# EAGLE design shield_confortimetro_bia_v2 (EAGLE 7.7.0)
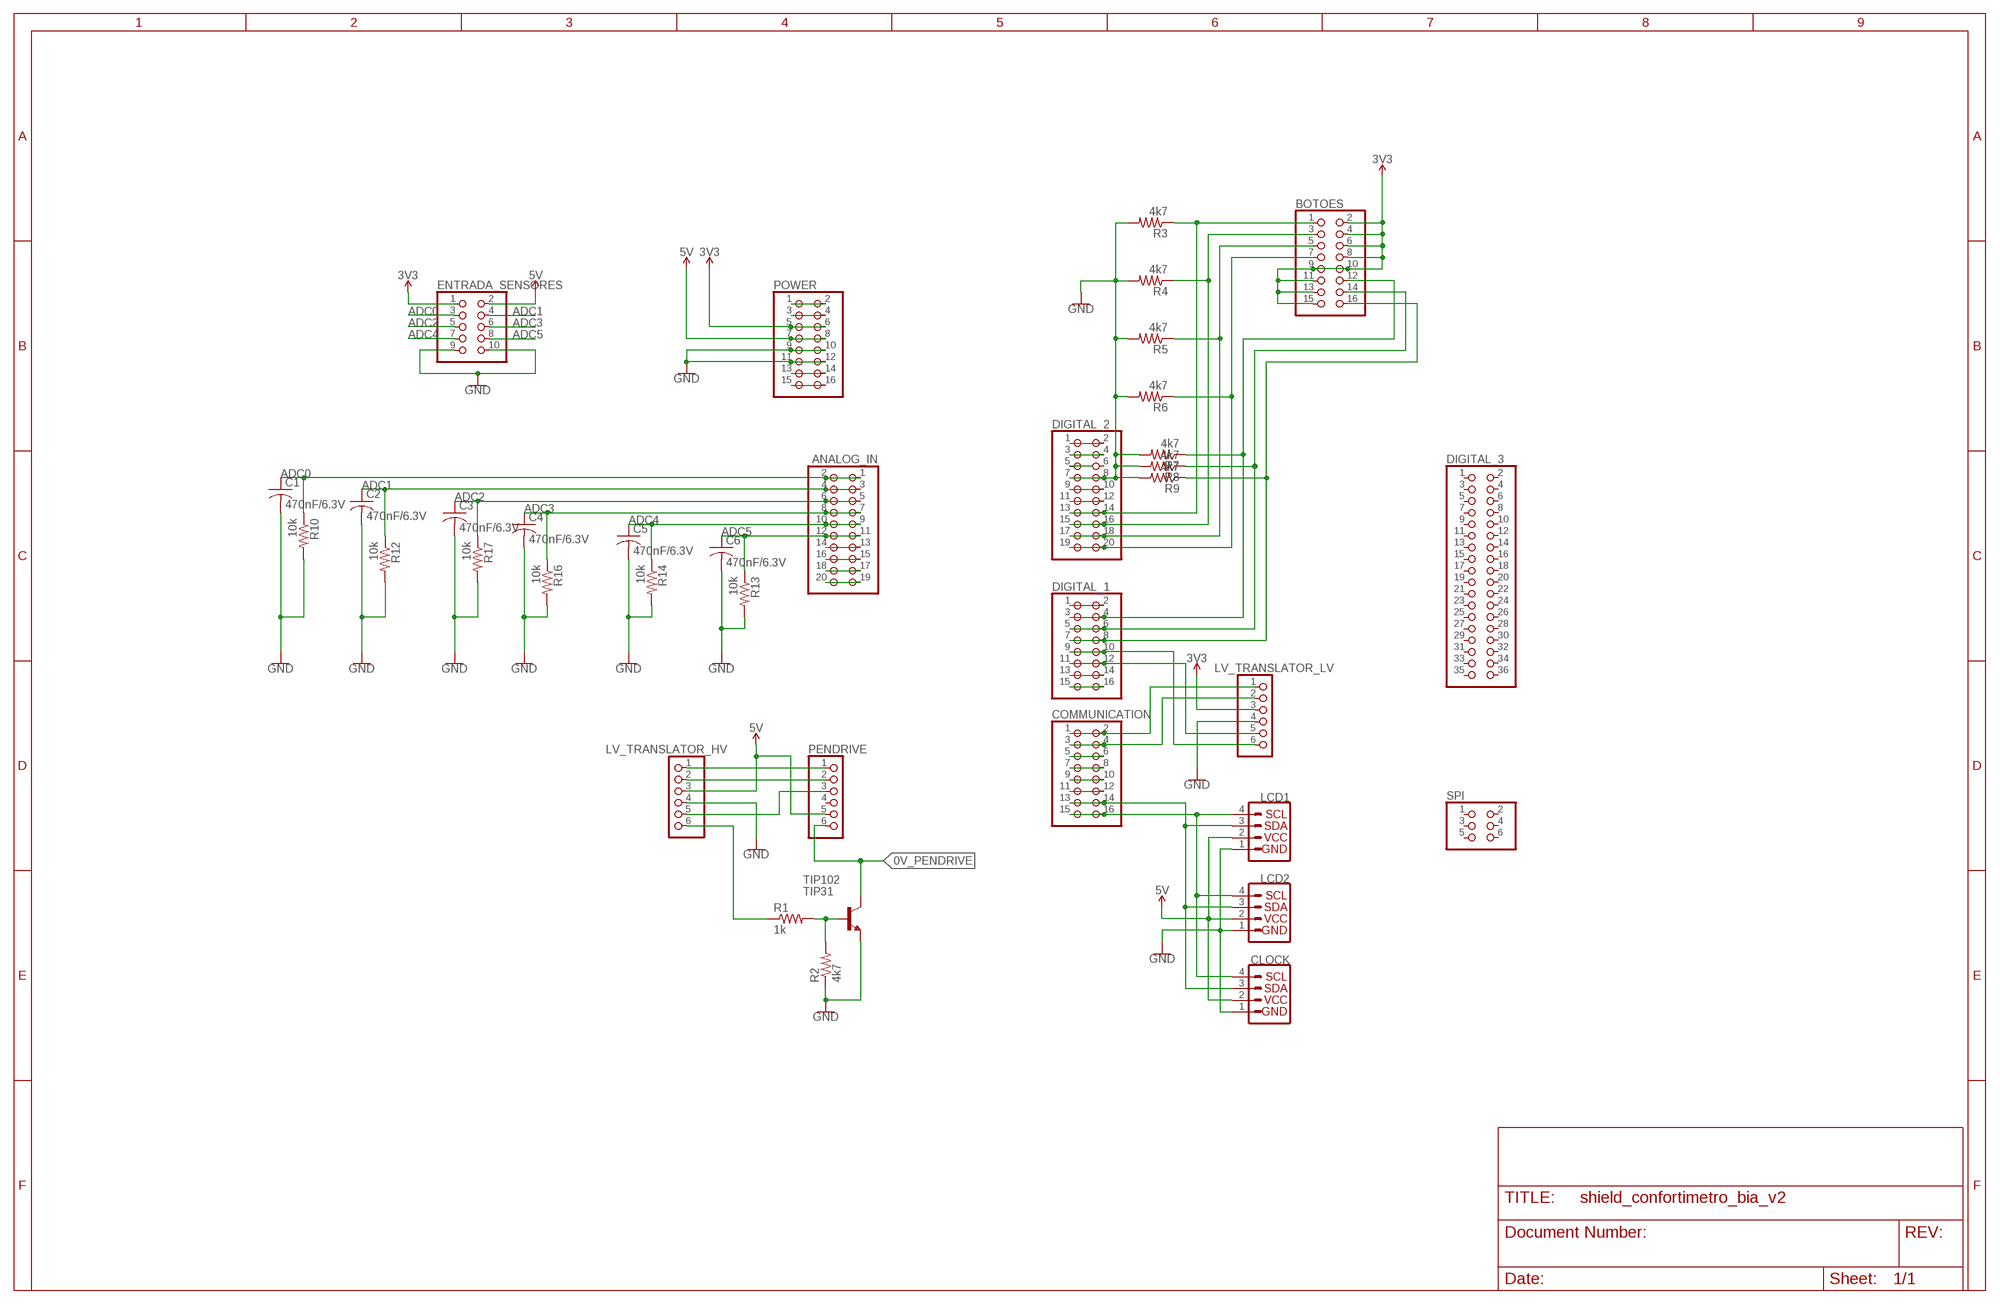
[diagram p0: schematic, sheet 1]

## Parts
ANALOG_IN  PINHD-2X10  [2X10]
BOTOES  PINHD-2X8  [2X08]
C1  470nF/6.3V  C-US050-030X075  [C050-030X075]
C2  470nF/6.3V  C-US050-030X075  [C050-030X075]
C3  470nF/6.3V  C-US050-030X075  [C050-030X075]
C4  470nF/6.3V  C-US050-030X075  [C050-030X075]
C5  470nF/6.3V  C-US050-030X075  [C050-030X075]
C6  470nF/6.3V  C-US050-030X075  [C050-030X075]
CLOCK  I2C_STANDARD  [1X04]
COMMUNICATION  PINHD-2X8  [2X08]
DIGITAL_1  PINHD-2X8  [2X08]
DIGITAL_2  PINHD-2X10  [2X10]
DIGITAL_3  PINHD-2X18  [2X18]
ENTRADA_SENSORES  PINHD-2X5  [2X05]
LCD1  I2C_STANDARD  [1X04]
LCD2  I2C_STANDARD  [1X04]
LV_TRANSLATOR_HV  PINHD-1X6  [1X06]
LV_TRANSLATOR_LV  PINHD-1X6  [1X06]
PENDRIVE  PINHD-1X6  [1X06]
POWER  PINHD-2X8  [2X08]
R1  1k  R-US_0309/12  [0309/12]
R2  4k7  R-US_0309/12  [0309/12]
R3  4k7  R-US_0309/12  [0309/12]
R4  4k7  R-US_0309/12  [0309/12]
R5  4k7  R-US_0309/12  [0309/12]
R6  4k7  R-US_0309/12  [0309/12]
R7  4k7  R-US_0309/12  [0309/12]
R8  4k7  R-US_0309/12  [0309/12]
R9  4k7  R-US_0309/12  [0309/12]
R10  10k  R-US_0309/12  [0309/12]
R12  10k  R-US_0309/12  [0309/12]
R13  10k  R-US_0309/12  [0309/12]
R14  10k  R-US_0309/12  [0309/12]
R16  10k  R-US_0309/12  [0309/12]
R17  10k  R-US_0309/12  [0309/12]
SPI  PINHD-2X3  [2X03]
TIP102  TIP31  [TO220]

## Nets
0V_PENDRIVE: PENDRIVE.6 TIP102.2(C)
ADC0: ANALOG_IN.1 ANALOG_IN.2 C1.1 ENTRADA_SENSORES.3 R10.1
ADC1: ANALOG_IN.3 ANALOG_IN.4 C2.1 ENTRADA_SENSORES.4 R12.1
ADC2: ANALOG_IN.5 ANALOG_IN.6 C3.1 ENTRADA_SENSORES.5 R17.1
ADC3: ANALOG_IN.7 ANALOG_IN.8 C4.1 ENTRADA_SENSORES.6 R16.1
ADC4: ANALOG_IN.9 ANALOG_IN.10 C5.1 ENTRADA_SENSORES.7 R14.1
ADC5: ANALOG_IN.11 ANALOG_IN.12 C6.1 ENTRADA_SENSORES.8 R13.1
GND: C1.2 C2.2 C3.2 C4.2 C5.2 C6.2 CLOCK.1 DIGITAL_2.7 DIGITAL_2.8 ENTRADA_SENSORES.9 ENTRADA_SENSORES.10 LCD1.1 LCD2.1 LV_TRANSLATOR_HV.4 LV_TRANSLATOR_LV.4 POWER.9 POWER.10 POWER.11 POWER.12 R2.1 R3.2 R4.2 R5.2 R6.2 R7.2 R8.2 R9.2 R10.2 R12.2 R13.2 R14.2 R16.2 R17.2 TIP102.3(E)
N$1: CLOCK.3 COMMUNICATION.13 COMMUNICATION.14 LCD1.3 LCD2.3
N$2: CLOCK.4 COMMUNICATION.15 COMMUNICATION.16 LCD1.4 LCD2.4
N$3: COMMUNICATION.1 COMMUNICATION.2 LV_TRANSLATOR_LV.1
N$4: COMMUNICATION.3 COMMUNICATION.4 LV_TRANSLATOR_LV.2
N$5: DIGITAL_1.9 DIGITAL_1.10 LV_TRANSLATOR_LV.6
N$6: DIGITAL_1.11 DIGITAL_1.12 LV_TRANSLATOR_LV.5
N$7: LV_TRANSLATOR_HV.1 PENDRIVE.1
N$8: LV_TRANSLATOR_HV.2 PENDRIVE.2
N$9: LV_TRANSLATOR_HV.5 PENDRIVE.3
N$10: R1.2 R2.2 TIP102.1(B)
N$11: LV_TRANSLATOR_HV.6 R1.1
N$12: BOTOES.12 DIGITAL_1.3 DIGITAL_1.4 R7.1
N$13: BOTOES.14 DIGITAL_1.5 DIGITAL_1.6 R8.1
N$14: BOTOES.16 DIGITAL_1.7 DIGITAL_1.8 R9.1
N$15: BOTOES.7 DIGITAL_2.19 DIGITAL_2.20 R6.1
N$16: BOTOES.5 DIGITAL_2.17 DIGITAL_2.18 R5.1
N$17: BOTOES.3 DIGITAL_2.15 DIGITAL_2.16 R4.1
N$18: BOTOES.1 DIGITAL_2.13 DIGITAL_2.14 R3.1
N$19: POWER.1 POWER.2
N$20: POWER.3 POWER.4
N$21: POWER.13 POWER.14
N$22: POWER.15 POWER.16
N$23: ANALOG_IN.13 ANALOG_IN.14
N$24: ANALOG_IN.15 ANALOG_IN.16
N$25: DIGITAL_2.1 DIGITAL_2.2
N$26: DIGITAL_2.3 DIGITAL_2.4
N$27: DIGITAL_2.5
N$29: DIGITAL_2.9 DIGITAL_2.10
N$30: DIGITAL_2.11 DIGITAL_2.12
N$31: DIGITAL_1.1 DIGITAL_1.2
N$32: DIGITAL_1.13 DIGITAL_1.14
N$33: DIGITAL_1.15 DIGITAL_1.16
N$34: COMMUNICATION.5 COMMUNICATION.6
N$35: COMMUNICATION.7 COMMUNICATION.8
N$36: COMMUNICATION.9 COMMUNICATION.10
N$37: COMMUNICATION.11 COMMUNICATION.12
N$38: ANALOG_IN.17 ANALOG_IN.18
N$39: ANALOG_IN.19 ANALOG_IN.20
VCC_3V3: BOTOES.2 BOTOES.4 BOTOES.6 BOTOES.8 BOTOES.9 BOTOES.10 BOTOES.11 BOTOES.13 BOTOES.15 ENTRADA_SENSORES.1 LV_TRANSLATOR_LV.3 POWER.5 POWER.6 ; supply symbol labelled 3V3
VCC_5V: CLOCK.2 ENTRADA_SENSORES.2 LCD1.2 LCD2.2 LV_TRANSLATOR_HV.3 PENDRIVE.5 POWER.7 POWER.8 ; supply symbol labelled 5V
Unconnected: DIGITAL_2.6 DIGITAL_3.1 DIGITAL_3.2 DIGITAL_3.3 DIGITAL_3.4 DIGITAL_3.5 DIGITAL_3.6 DIGITAL_3.7 DIGITAL_3.8 DIGITAL_3.9 DIGITAL_3.10 DIGITAL_3.11 DIGITAL_3.12 DIGITAL_3.13 DIGITAL_3.14 DIGITAL_3.15 DIGITAL_3.16 DIGITAL_3.17 DIGITAL_3.18 DIGITAL_3.19 DIGITAL_3.20 DIGITAL_3.21 DIGITAL_3.22 DIGITAL_3.23 DIGITAL_3.24 DIGITAL_3.25 DIGITAL_3.26 DIGITAL_3.27 DIGITAL_3.28 DIGITAL_3.29 DIGITAL_3.30 DIGITAL_3.31 DIGITAL_3.32 DIGITAL_3.33 DIGITAL_3.34 DIGITAL_3.35 DIGITAL_3.36 PENDRIVE.4 SPI.1 SPI.2 SPI.3 SPI.4 SPI.5 SPI.6

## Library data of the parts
ANALOG_IN = SparkFun-Retired:PINHD-2X10: PIN HEADER
BOTOES COMMUNICATION DIGITAL_1 POWER = pinhead:PINHD-2X8: PIN HEADER
C1-C6 = adafruit:C-US: CAPACITOR, American symbol
CLOCK LCD1 LCD2 = SparkFun-Connectors:I2C_STANDARD: SparkFun I2C Standard Pinout Header SparkFun has standardized on a pinout for all I2C based sensor breakouts. This pinout allows I2C boards to be plugged directly into the headers on Arduino Uno compatible boards, and to be daisy chained easily. Example SparkFun Products: SparkFun Atmospheric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
DIGITAL_2 = pinhead:PINHD-2X10: PIN HEADER
DIGITAL_3 = pinhead:PINHD-2X18: PIN HEADER
ENTRADA_SENSORES = pinhead:PINHD-2X5: PIN HEADER
LV_TRANSLATOR_HV LV_TRANSLATOR_LV PENDRIVE = adafruit:PINHD-1X6: PIN HEADER
R1-R10 R12-R14 R16 R17 = adafruit:R-US_: RESISTOR, American symbol
SPI = pinhead:PINHD-2X3: PIN HEADER
TIP102 = transistor:TIP31: NPN Transistor Medium Power Linear Switching Applications Source: http://onsemi.com

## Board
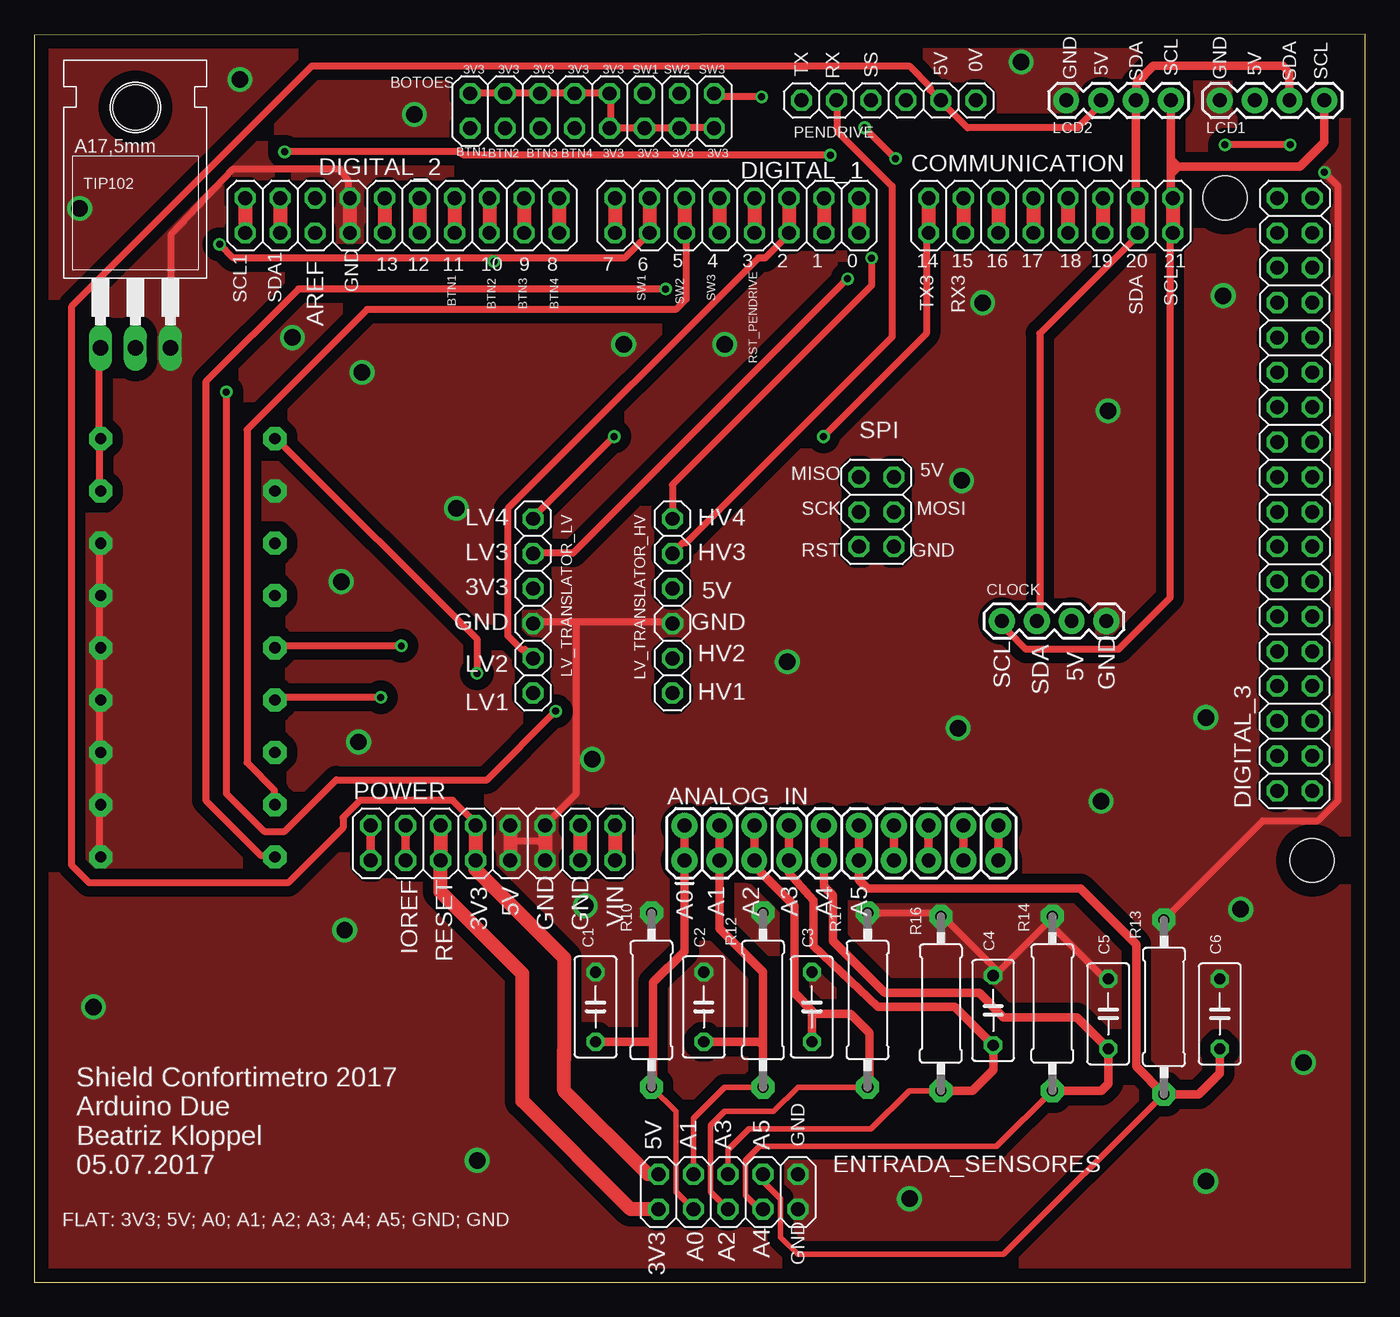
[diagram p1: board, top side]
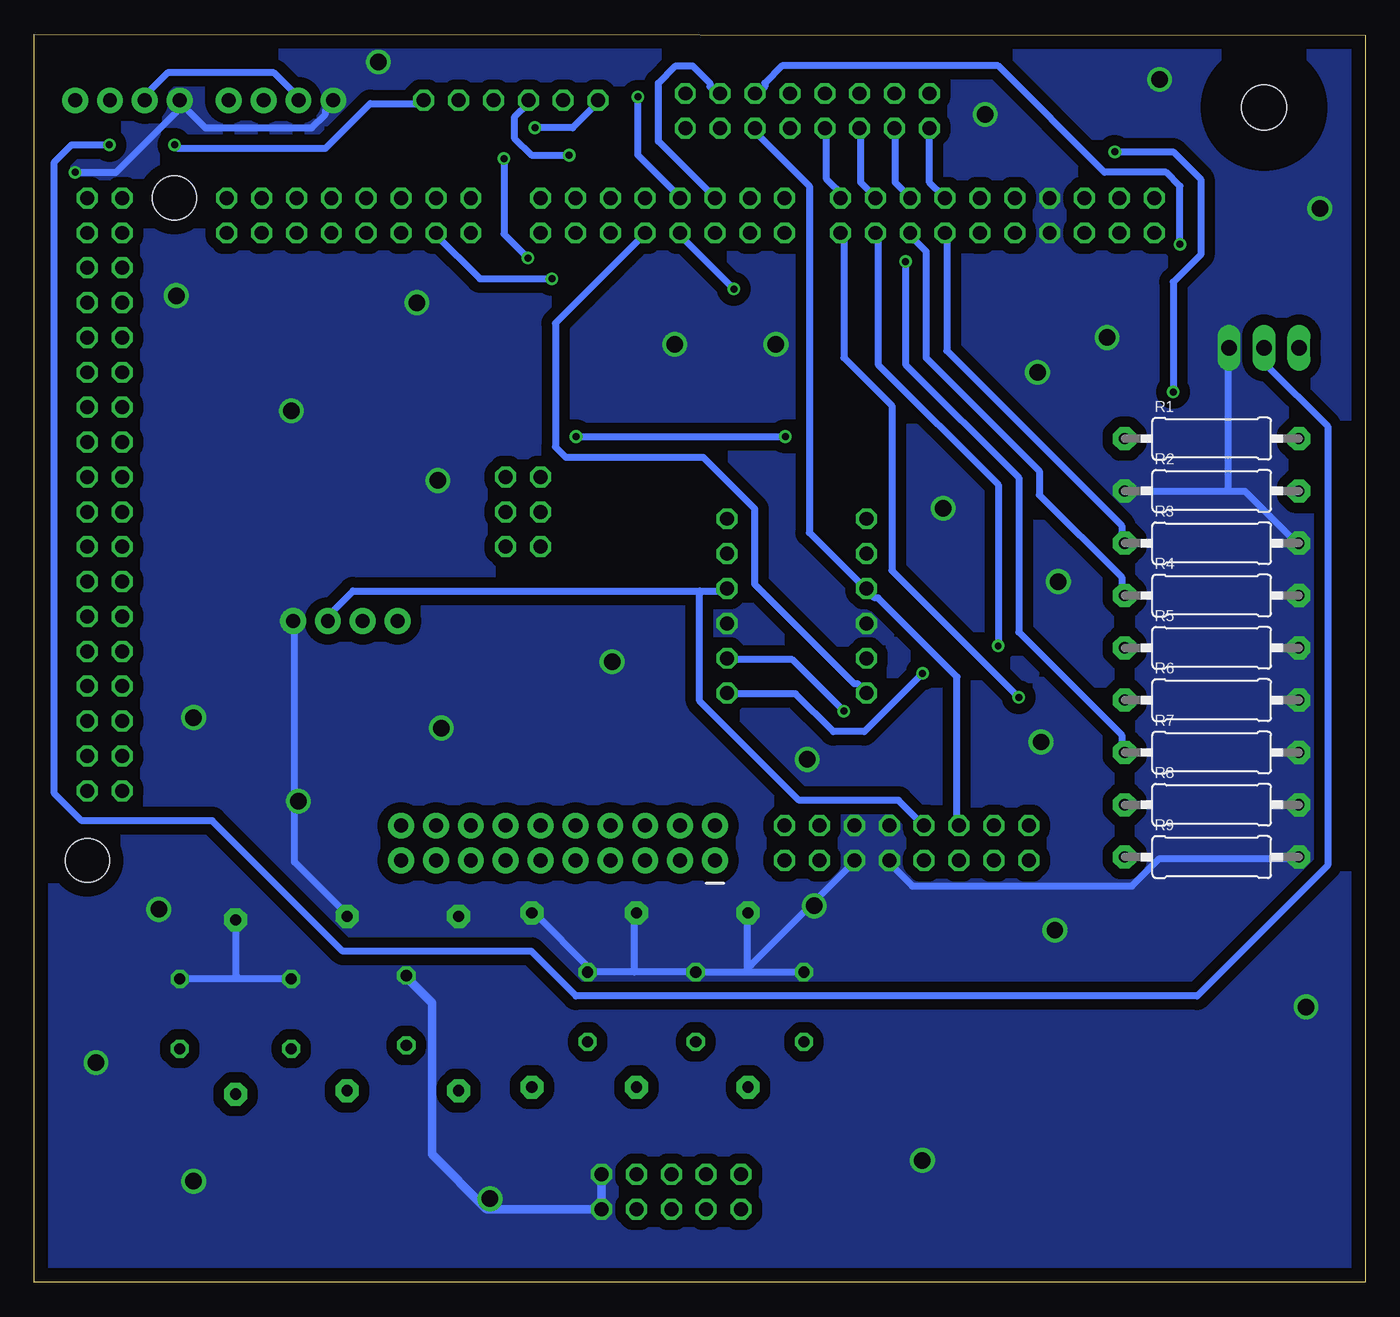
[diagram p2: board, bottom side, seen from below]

Size 96.95 x 90.92 mm. Coordinates in mm from the lower left corner, seen from the top.
Outline: 0,0 96.95,0 96.95,90.92 0,90.86 0,0
Copper layers (1*16): Top 0.035mm / dielectric 1.5mm / Bottom 0.035mm
Design rules "default *": minimum track width 20mil, minimum drill 20mil, track to track 30mil, track to pad 30mil, pad to pad 30mil, via to via 30mil, smd to smd 8mil, copper to edge 40mil, drill to drill 10mil, minimum pad ring 10mil, minimum via ring 8mil, stop-mask expansion 4mil, vias tented up to drill 0mil, thermal gap 10mil
Holes 3.2 mm at 93.09,30.73 86.74,78.99

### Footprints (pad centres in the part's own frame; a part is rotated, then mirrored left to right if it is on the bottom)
2X10 = drill 1.016 pad 1.88: 1 0,0; 2 0,2.54; 3 2.54,0; 4 2.54,2.54; 5 5.08,0; 6 5.08,2.54; 7 7.62,0; 8 7.62,2.54; 9 10.16,0; 10 10.16,2.54; 11 12.7,0; 12 12.7,2.54; 13 15.24,0; 14 15.24,2.54; 15 17.78,0; 16 17.78,2.54; 17 20.32,0; 18 20.32,2.54; 19 22.86,0; 20 22.86,2.54
2X08 = drill 1.016 octagon: 1 -8.89,-1.27; 2 -8.89,1.27; 3 -6.35,-1.27; 4 -6.35,1.27; 5 -3.81,-1.27; 6 -3.81,1.27; 7 -1.27,-1.27; 8 -1.27,1.27; 9 1.27,-1.27; 10 1.27,1.27; 11 3.81,-1.27; 12 3.81,1.27; 13 6.35,-1.27; 14 6.35,1.27; 15 8.89,-1.27; 16 8.89,1.27
C050-030X075 = drill 0.813 octagon: 1 -2.54,0; 2 2.54,0
1X04 = drill 1.016 pad 1.88: 1 0,0; 2 2.54,0; 3 5.08,0; 4 7.62,0
2X10' = drill 1.016 octagon: 1 -11.43,-1.27; 2 -11.43,1.27; 3 -8.89,-1.27; 4 -8.89,1.27; 5 -6.35,-1.27; 6 -6.35,1.27; 7 -3.81,-1.27; 8 -3.81,1.27; 9 -1.27,-1.27; 10 -1.27,1.27; 11 1.27,-1.27; 12 1.27,1.27; 13 3.81,-1.27; 14 3.81,1.27; 15 6.35,-1.27; 16 6.35,1.27; 17 8.89,-1.27; 18 8.89,1.27; 19 11.43,-1.27; 20 11.43,1.27
2X18 = drill 1.016 octagon: 1 -21.59,-1.27; 2 -21.59,1.27; 3 -19.05,-1.27; 4 -19.05,1.27; 5 -16.51,-1.27; 6 -16.51,1.27; 7 -13.97,-1.27; 8 -13.97,1.27; 9 -11.43,-1.27; 10 -11.43,1.27; 11 -8.89,-1.27; 12 -8.89,1.27; 13 -6.35,-1.27; 14 -6.35,1.27; 15 -3.81,-1.27; 16 -3.81,1.27; 17 -1.27,-1.27; 18 -1.27,1.27; 19 1.27,-1.27; 20 1.27,1.27; 21 3.81,-1.27; 22 3.81,1.27; 23 6.35,-1.27; 24 6.35,1.27; 25 8.89,-1.27; 26 8.89,1.27; 27 11.43,-1.27; 28 11.43,1.27; 29 13.97,-1.27; 30 13.97,1.27; 31 16.51,-1.27; 32 16.51,1.27; 33 19.05,-1.27; 34 19.05,1.27; 35 21.59,-1.27; 36 21.59,1.27
2X05 = drill 1.016 octagon: 1 -5.08,-1.27; 2 -5.08,1.27; 3 -2.54,-1.27; 4 -2.54,1.27; 5 0,-1.27; 6 0,1.27; 7 2.54,-1.27; 8 2.54,1.27; 9 5.08,-1.27; 10 5.08,1.27
1X06 = drill 1.016 octagon: 1 -6.35,0; 2 -3.81,0; 3 -1.27,0; 4 1.27,0; 5 3.81,0; 6 6.35,0
0309/12 = drill 0.813 pad 1.676 octagon: 1 -6.35,0; 2 6.35,0
2X03 = drill 1.016 octagon: 1 -2.54,-1.27; 2 -2.54,1.27; 3 0,-1.27; 4 0,1.27; 5 2.54,-1.27; 6 2.54,1.27
TO220 = drill 1.118 long: 1 -2.54,-6.35; 2 0,-6.35; 3 2.54,-6.35 | hole 3.302: 0,11.176

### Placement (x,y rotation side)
ANALOG_IN  47.37,30.73 0 top
BOTOES  40.64,85.34 0 top
C1  40.89,20.07 90 top
C2  48.77,20.07 90 top
C3  56.64,20.07 90 top
C4  69.85,19.81 90 top
C5  78.23,19.56 90 top
C6  86.36,19.56 90 top
CLOCK  78.11,48.18 180 top
COMMUNICATION  74.04,77.72 0 top
DIGITAL_1  51.18,77.72 0 top
DIGITAL_2  [2X10']  26.8,77.72 0 top
DIGITAL_3  91.82,57.4 90 top
ENTRADA_SENSORES  50.55,6.6 0 top
LCD1  86.36,86.11 0 top
LCD2  75.17,86.11 0 top
LV_TRANSLATOR_HV  46.48,49.28 270 top
LV_TRANSLATOR_LV  36.32,49.28 270 top
PENDRIVE  62.23,86.11 0 top
POWER  33.4,32 0 top
R1  11.18,61.47 0 bottom
R2  11.18,57.66 0 bottom
R3  11.18,53.85 0 bottom
R4  11.18,50.04 0 bottom
R5  11.18,46.23 0 bottom
R6  11.18,42.42 0 bottom
R7  11.18,38.61 0 bottom
R8  11.18,34.8 0 bottom
R9  11.18,30.99 0 bottom
R10  44.96,20.57 90 top
R12  53.09,20.57 90 top
R13  82.3,20.07 90 top
R14  74.17,20.32 90 top
R16  66.04,20.32 90 top
R17  60.71,20.57 90 top
SPI  61.34,56.13 90 top
TIP102  7.37,74.42 0 top

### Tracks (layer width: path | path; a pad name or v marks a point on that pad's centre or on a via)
0V_PENDRIVE  (via drill 0.51)
  Top 0.508: v91.49,82.87 v86.74,82.87
  Bottom 0.508: v86.74,82.87 86.49,82.62 75.74,82.62 72.49,85.87 68.74,85.87 PENDRIVE.6 | v91.49,82.87 94.24,82.87 95.49,81.62 95.49,35.62 93.49,33.62 83.99,33.62 74.49,24.12 60.74,24.12 57.49,20.87 12.24,20.87 2.74,30.37 2.74,62.37 7.24,66.87 7.24,67.87 TIP102.2
ADC0
  Top 0.406: ENTRADA_SENSORES.3 46.74,6.6 46.74,12.45 R10.1
  Top 0.61: 45.09,17.53 45.09,21.84 47.37,24.13 ANALOG_IN.1 ANALOG_IN.2 | 45.09,17.53 45.09,14.35 R10.1 | C1.1 45.09,17.53
ADC1
  Top 0.406: ENTRADA_SENSORES.4 48.01,11.94 50.29,14.22 R12.1
  Top 0.61: 53.09,17.27 53.09,22.61 49.91,25.78 ANALOG_IN.3 ANALOG_IN.4 | 53.09,17.27 R12.1 | C2.1 52.83,17.53 53.09,17.27
ADC2
  Top 0.406: R17.1 55.63,14.22 53.85,12.45 50.29,12.45 49.28,11.43 49.28,6.6 ENTRADA_SENSORES.5
  Top 0.61: 56.77,19.68 55.37,21.08 55.37,27.43 52.45,30.35 ANALOG_IN.5 ANALOG_IN.6 | 56.77,19.68 56.9,19.56 59.44,19.56 60.83,18.16 60.83,14.35 R17.1 | C3.1 56.64,19.56 56.77,19.68
ADC3
  Top 0.406: ENTRADA_SENSORES.6 50.55,9.65 52.07,11.18 60.96,11.18 63.75,13.97 R16.1
  Top 0.61: R16.1 68.33,13.97 69.85,15.49 C4.1 67.06,20.07 61.47,20.07 56.77,24.51 56.77,27.81 54.99,29.84 ANALOG_IN.7 ANALOG_IN.8
ADC4
  Top 0.406: ENTRADA_SENSORES.7 52.83,5.33 51.82,6.35 51.82,8.89 52.83,9.91 70.1,9.91 R14.1
  Top 0.61: R14.1 77.72,13.97 78.23,14.48 C5.1 75.95,19.3 70.61,19.3 68.83,21.08 61.98,21.08 58.17,24.89 58.17,28.19 57.53,28.83 ANALOG_IN.9 ANALOG_IN.10
ADC5
  Top 0.406: ENTRADA_SENSORES.8 53.09,7.37 54.36,6.1 54.36,3.3 55.63,2.03 70.61,2.03 R13.1
  Top 0.61: C6.1 86.36,15.24 84.84,13.72 R13.1 80.26,15.75 80.26,24.64 76.2,28.7 60.71,28.7 60.07,29.34 ANALOG_IN.11 ANALOG_IN.12
GND  (via drill 0.51, 1.2)
  Top 0.508: TIP102.3 9.99,68.12 9.99,76.37 14.49,81.12 22.26,81.12 22.86,80.26 22.86,78.99 | R9.2 4.74,31.12 4.74,34.62 R8.2 4.74,34.87 4.74,38.37 R7.2 4.74,38.62 4.74,42.37 R6.2 4.74,42.62 4.74,46.12 R5.2 4.74,46.37 4.74,49.87 R4.2 4.74,50.12 4.74,53.62 R3.2 | 39.49,48.12 46.24,48.12 LV_TRANSLATOR_HV.4 | 39.49,48.12 36.49,48.12 LV_TRANSLATOR_LV.4 | R17.2 60.74,26.87 65.99,26.87 R16.2 66.24,26.62 70.24,22.62 | 34.67,32.12 34.99,32.12 36.74,32.12 37.21,32.12 | 39.49,48.12 39.49,47.87 39.49,35.62 37.49,33.62 POWER.12 | 70.24,22.62 74.24,26.62 R14.2 73.99,26.12 77.99,22.12 C5.2 | 70.24,22.62 69.99,22.37 C4.2 70.24,22.62 | v93.99,80.87 94.99,79.87 94.99,35.12 93.49,33.62 89.49,33.62 82.49,26.62 R13.2
  Top 1.016: POWER.10 34.67,32.12 POWER.9 | POWER.12 37.21,32.12 POWER.11 | DIGITAL_2.8 DIGITAL_2.7
  Bottom 0.508: 9.99,57.62 8.74,57.62 4.99,53.87 R3.2 | 9.99,57.62 17.49,57.62 R2.1 | TIP102.3 9.99,67.87 9.99,57.87 9.99,57.62 | 44.99,22.62 48.74,22.62 C2.2 48.99,22.62 53.24,22.62 | 44.99,22.62 40.99,22.62 C1.2 | 53.24,22.62 56.49,22.62 C3.2 56.49,22.87 60.49,26.87 R17.2 | 44.99,23.12 44.99,22.87 44.99,22.62 | 44.99,23.12 44.99,26.87 R10.2 | R12.2 53.24,26.87 53.24,22.87 53.24,22.62 | POWER.11 37.24,30.62 44.74,23.12 44.99,23.12 | LCD2.1 75.24,85.87 75.74,85.37 75.74,85.12 76.74,84.12 84.49,84.12 86.24,85.87 LCD1.1 86.24,85.62 90.99,80.87 v93.99,80.87 | 82.24,22.12 78.24,22.12 C5.2 | 82.24,22.12 86.24,22.12 C6.2 | R13.2 82.24,26.37 82.24,22.37 82.24,22.12 | CLOCK.1 77.99,48.12 77.99,30.62 74.24,26.87 R14.2 | 69.74,22.12 C4.2 | R9.2 4.99,30.87 14.99,30.87 16.99,28.87 32.99,28.87 34.74,30.62 POWER.9
  Bottom 0.61: 69.74,22.12 67.99,20.37 67.99,10.37 67.99,9.31 64.01,5.33 ENTRADA_SENSORES.9 ENTRADA_SENSORES.10
  other vias: 71.88,88.9 67.56,58.42 69.09,71.37 78.23,63.5 86.61,71.88 85.34,41.15 54.86,45.21 67.31,40.39 77.72,35.05 87.88,27.18 85.34,7.37 92.46,16 32.26,8.89 4.32,20.07 22.61,25.65 23.62,39.37 22.35,51.05 23.88,66.29 27.69,85.09 14.99,87.63 30.73,56.39 50.29,68.33 40.64,38.1 40.13,27.43 3.3,78.23 42.93,68.33 18.8,68.83 63.75,6.1
  pour Top (isolate 0.305, no thermals): 0,90.93 0,0 97.03,0 97.03,4.06 97.28,4.06 97.28,90.93
  pour Bottom (isolate 0.406, rank 2, no thermals): 0,90.93 0,0 97.03,0 97.03,4.06 97.28,4.06 97.28,90.93
N$1
  Top 0.508: CLOCK.3 73.24,48.37 73.24,69.12 80.24,76.12 COMMUNICATION.13
  Top 0.61: LCD1.3 91.44,88.14 90.93,88.65 81.53,88.65 80.26,87.38 80.26,86.12 LCD2.3 80.25,78.99 COMMUNICATION.14
  Top 1.016: COMMUNICATION.14 COMMUNICATION.13
N$2
  Top 0.508: CLOCK.4 70.49,48.12 70.99,47.62 70.99,47.37 72.24,46.12 78.99,46.12 82.74,49.87 82.74,76.12 COMMUNICATION.15
  Top 0.61: LCD1.4 93.98,83.06 92.46,81.53 92.2,81.28 83.57,81.28 | COMMUNICATION.16 83.06,79.12 82.79,79.12 82.79,81.28 | 83.31,81.28 82.93,81.28 82.79,81.28 | 83.31,81.28 83.57,81.28 | 82.79,81.28 LCD2.4 | 82.8,80.77 83.31,81.28 | 83.57,81.28 83.31,81.28 | 83.31,81.28 82.8,81.79
  Top 1.016: COMMUNICATION.16 COMMUNICATION.15
N$3  (via drill 0.51)
  Top 0.508: v42.24,61.62 36.49,55.87 LV_TRANSLATOR_LV.1 | v57.49,61.62 64.99,69.12 64.99,76.12 COMMUNICATION.1
  Top 1.016: COMMUNICATION.2 COMMUNICATION.1
  Bottom 0.508: v57.49,61.62 v42.24,61.62
N$4  (via drill 0.51)
  Top 0.508: v59.24,73.12 39.24,53.12 36.49,53.12 LV_TRANSLATOR_LV.2
  Top 1.016: COMMUNICATION.4 COMMUNICATION.3
  Bottom 0.508: v59.24,73.12 64.49,73.12 67.74,76.37 COMMUNICATION.3
N$5
  Top 1.016: DIGITAL_1.10 DIGITAL_1.9
  Bottom 0.508: LV_TRANSLATOR_LV.6 36.49,43.12 36.99,43.62 37.24,43.62 44.49,50.87 44.49,56.37 48.24,60.12 58.24,60.12 58.99,60.87 58.99,69.87 52.49,76.37 DIGITAL_1.9
N$6
  Top 0.508: LV_TRANSLATOR_LV.5 36.24,45.62 35.74,46.12 35.49,46.12 34.49,47.12 34.49,56.37 52.74,74.62 53.24,74.62 54.74,76.12 DIGITAL_1.11
  Top 1.016: DIGITAL_1.12 DIGITAL_1.11
N$7  (via drill 0.51)
  Top 0.508: v60.99,74.62 60.99,72.62 46.49,58.12 46.49,55.87 LV_TRANSLATOR_HV.1 | v60.49,84.12 v62.74,81.87
  Bottom 0.508: v60.99,74.62 62.74,76.37 v62.74,81.87 | v60.49,84.12 57.74,84.12 55.99,85.87 PENDRIVE.1
N$8
  Top 0.508: LV_TRANSLATOR_HV.2 46.49,53.12 47.24,53.87 47.49,53.87 62.49,68.87 62.49,79.87 58.49,83.87 58.49,85.87 PENDRIVE.2
N$9  (via drill 0.51)
  Top 0.508: v37.99,41.62 32.99,36.62 21.99,36.62 18.24,32.87 16.74,32.87 13.99,35.62 v13.99,64.87 | v18.24,82.37 30.99,82.37 31.24,82.12 v57.99,82.12
  Bottom 0.508: v37.99,41.62 41.74,45.37 46.24,45.37 LV_TRANSLATOR_HV.5 | v13.99,64.87 13.99,72.87 11.99,74.87 11.99,80.37 13.99,82.37 v18.24,82.37 | v57.99,82.12 60.74,82.12 61.99,83.37 61.99,84.87 60.99,85.87 PENDRIVE.3
N$10
  Top 0.508: R2.2 4.74,57.87 4.74,61.37 R1.2 4.74,61.62 4.74,67.87 TIP102.1
N$11  (via drill 0.51)
  Top 0.508: v32.24,44.37 32.24,46.87 17.74,61.37 R1.1
  Bottom 0.508: v32.24,44.37 36.49,40.12 38.74,40.12 41.49,42.87 46.24,42.87 LV_TRANSLATOR_HV.6
N$12  (via drill 0.51)
  Top 0.508: v13.49,75.62 14.49,74.62 33.49,74.62 | 33.49,74.62 42.99,74.62 44.49,76.12 DIGITAL_1.3 | v33.49,74.37 33.49,74.62
  Top 1.016: DIGITAL_1.4 DIGITAL_1.3
  Bottom 0.508: v13.49,75.62 13.49,79.87 14.49,80.87 18.99,80.87 26.74,88.62 42.49,88.62 43.74,87.37 43.74,87.12 44.24,86.62 BOTOES.12 | v33.49,74.37 33.49,66.87 25.24,58.62 25.24,47.37 17.74,39.87 17.74,38.62 R7.1
N$13
  Top 0.508: R8.1 17.49,34.87 17.49,35.87 15.49,37.87 15.49,62.12 24.24,70.87 46.74,70.87 47.49,71.62 47.49,76.12 DIGITAL_1.5
  Top 1.016: DIGITAL_1.6 DIGITAL_1.5
  Bottom 0.508: BOTOES.14 47.24,86.62 47.74,87.12 47.74,87.37 48.99,88.62 50.24,88.62 51.49,87.37 51.49,83.12 47.49,79.12 DIGITAL_1.6
N$14  (via drill 0.51)
  Top 0.508: v52.99,86.37 49.74,86.37 BOTOES.16 | v45.99,72.37 19.24,72.37 12.49,65.62 12.49,35.12 16.49,31.12 17.49,31.12 R9.1
  Top 1.016: DIGITAL_1.8 DIGITAL_1.7
  Bottom 0.508: v52.99,86.37 52.99,82.12 49.99,79.12 DIGITAL_1.8 | v45.99,72.37 49.99,76.37 DIGITAL_1.7
N$15  (via drill 0.51)
  Top 0.508: v25.24,42.62 17.74,42.62 R6.1
  Top 1.016: DIGITAL_2.20 DIGITAL_2.19
  Bottom 0.508: BOTOES.7 39.24,83.87 39.24,80.37 37.99,79.12 DIGITAL_2.20 | v25.24,42.62 34.49,51.87 34.49,63.87 37.99,67.37 37.99,76.37 DIGITAL_2.19
N$16  (via drill 0.51)
  Top 0.508: v26.74,46.37 17.74,46.37 R5.1
  Top 1.016: DIGITAL_2.18 DIGITAL_2.17
  Bottom 0.508: BOTOES.5 36.74,83.87 36.74,80.12 35.74,79.12 DIGITAL_2.18 | v26.74,46.37 26.74,58.12 35.49,66.87 35.49,76.37 DIGITAL_2.17
N$17
  Top 1.016: DIGITAL_2.16 DIGITAL_2.15
  Bottom 0.508: BOTOES.3 34.24,83.87 34.24,80.12 33.24,79.12 DIGITAL_2.16 | R4.1 17.74,50.12 17.74,51.37 23.74,57.37 23.74,59.12 31.99,67.37 31.99,75.12 33.24,76.37 DIGITAL_2.15
N$18
  Top 1.016: DIGITAL_2.14 DIGITAL_2.13
  Bottom 0.508: BOTOES.1 31.74,83.87 31.74,80.12 30.74,79.12 DIGITAL_2.14 | R3.1 17.74,53.87 17.74,55.12 30.49,67.87 30.49,76.37 DIGITAL_2.13
N$19
  Top 0.61: POWER.2 POWER.1
N$20
  Top 0.61: POWER.4 POWER.3
N$21
  Top 1.016: POWER.14 POWER.13
N$22
  Top 1.016: POWER.16 POWER.15
N$23
  Top 0.61: ANALOG_IN.14 ANALOG_IN.13
N$24
  Top 0.61: ANALOG_IN.16 ANALOG_IN.15
N$25
  Top 1.016: DIGITAL_2.2 DIGITAL_2.1
N$26
  Top 1.016: DIGITAL_2.4 DIGITAL_2.3
N$29
  Top 1.016: DIGITAL_2.10 DIGITAL_2.9
N$30
  Top 1.016: DIGITAL_2.12 DIGITAL_2.11
N$31
  Top 1.016: DIGITAL_1.2 DIGITAL_1.1
N$32
  Top 1.016: DIGITAL_1.14 DIGITAL_1.13
N$33
  Top 1.016: DIGITAL_1.16 DIGITAL_1.15
N$34
  Top 1.016: COMMUNICATION.6 COMMUNICATION.5
N$35
  Top 1.016: COMMUNICATION.8 COMMUNICATION.7
N$36
  Top 1.016: COMMUNICATION.10 COMMUNICATION.9
N$37
  Top 1.016: COMMUNICATION.12 COMMUNICATION.11
N$38
  Top 0.61: ANALOG_IN.18 ANALOG_IN.17
N$39
  Top 0.61: ANALOG_IN.20 ANALOG_IN.19
VCC_3V3
  Top 0.508: BOTOES.2 31.99,86.62 34.24,86.62 BOTOES.4 34.49,86.62 36.74,86.62 BOTOES.6 36.99,86.62 39.24,86.62 BOTOES.8 39.49,86.62 41.74,86.62 BOTOES.10 41.99,86.37 41.99,84.12 BOTOES.9 42.24,84.12 44.24,84.12 BOTOES.11 44.49,84.12 46.74,84.12 BOTOES.13 47.24,84.12 49.49,84.12 BOTOES.15
  Top 1.016: 35.56,16 35.56,16.26 | 35.56,16.26 35.56,22.48 29.59,28.45 POWER.5 POWER.6 | ENTRADA_SENSORES.1 43.43,5.33 35.56,13.21 35.56,16.26
  Bottom 0.508: POWER.6 29.74,33.37 29.74,44.12 35.49,49.87 35.74,49.87 36.24,50.37 LV_TRANSLATOR_LV.3 36.49,50.62 40.49,54.62 40.49,79.87 44.49,83.87 BOTOES.11
VCC_5V
  Top 0.508: LCD2.2 77.74,85.87 75.99,84.12 67.99,84.12 66.24,85.87 PENDRIVE.5 65.99,86.12 65.24,86.87 65.24,87.12 63.74,88.62 20.24,88.62 2.74,71.12 2.74,30.37 3.99,29.12 18.49,29.12 22.49,33.12 22.49,33.87 23.74,35.12 30.49,35.12 31.99,33.62 POWER.8
  Top 1.016: 38.61,17.02 38.61,23.62 32.13,30.1 POWER.7 POWER.8 | 38.61,17.02 38.61,16.26 | ENTRADA_SENSORES.2 44.7,7.87 38.61,13.97 38.61,17.02
  Bottom 0.508: 48.49,50.37 73.74,50.37 75.74,48.37 CLOCK.2 | 48.49,50.37 46.49,50.37 LV_TRANSLATOR_HV.3 | LCD1.2 88.74,86.12 88.74,86.62 87.24,88.12 79.49,88.12 77.49,86.12 LCD2.2 | 48.49,50.37 48.49,50.12 48.49,42.37 41.24,35.12 33.99,35.12 32.24,33.37 POWER.8

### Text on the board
tNames: 0V | SDA | SDA | TX | RX | SS | 5V | 5V | 5V | 3V3 | 3V3 | 3V3 | 3V3 | 3V3 | SW1 | SW2 | SW3 | SCL | GND | GND | SCL | BTN1 | BTN2 | BTN3 | BTN4 | 3V3 | 3V3 | 3V3 | 3V3 | AREF | 5 | 4 | 3 | 2 | 1 | 0 | 14 | 15 | 16 | 17 | 18 | 19 | 20 | 21 | 13 | 12 | 11 | 10 | BTN2 | 9 | BTN3 | 8 | BTN4 | 7 | 6 | SW1 | SW2 | SW3 | RST_PENDRIVE | TX3 | RX3 | SDA | GND | SCL1 | SDA1 | BTN1 | SCL | MISO | 5V | LV4 | HV4 | SCK | MOSI | LV3 | HV3 | GND | RST | 3V3 | 5V | GND | GND | HV2 | SCL | SDA | 5V | LV2 | LV1 | HV1 | GND | 5V | VIN | A0 | A1 | A2 | A3 | A4 | A5 | 3V3 | GND | GND | IOREF | RESET | GND | 5V | A1 | A3 | A5 | Shield Confortimetro 2017 / Arduino Due / Beatriz Kloppel / 05.07.2017 | FLAT: 3V3; 5V; A0; A1; A2; A3; A4; A5; GND; GND | A0 | A2 | A4 | GND | 3V3

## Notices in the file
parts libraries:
SparkFun-Connectors: Licensing: Creative Commons ShareAlike 4.0 International - https://creativecommons.org/licenses/by-sa/4.0
